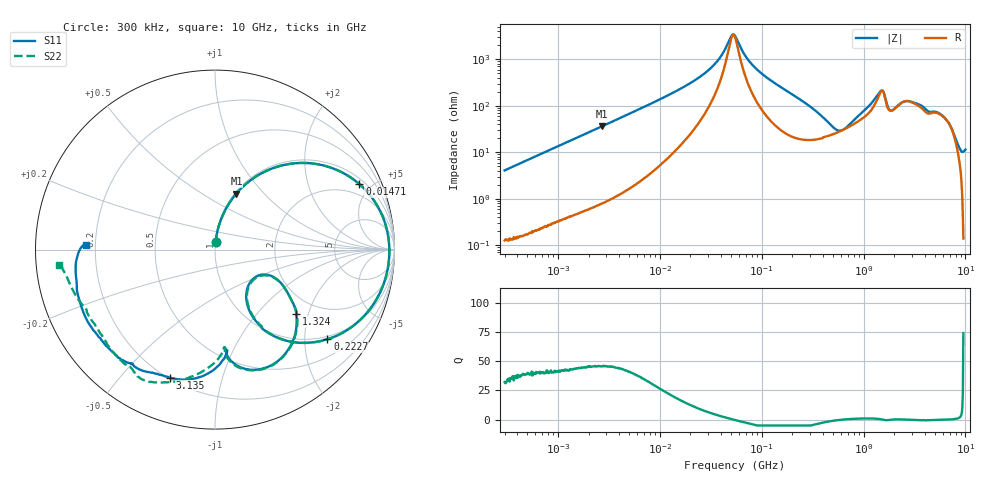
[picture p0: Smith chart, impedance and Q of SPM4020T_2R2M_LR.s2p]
! S-Parameter Data Generated by TDK Corporation
! Copyright(C) 2019 TDK Corporation.
! All Rights Reserved.
! TDK P/N: SPM4020T-2R2M-LR (Inductor)
! Property: L=2.2uH at 100kHz
! Size(LxWxT): 4.4x4.1x2mm
! Model Type: s2p (Touchstone File Format Version 1.0)
! Frequency: DC=Yes Start=0.3MHz Stop=10000MHz 802points Log-sweep
! Model Generated on Sep. 23, 2019
! Port Assignments:
!  1 ---@@@--- 2
! Applicable Conditions:
!  Temperature = 25 degC
!  DC Bias Current = 0 A
!  Small Signal Operation
! Terms and conditions regarding TDK Simulation Models
! (1)This simulation model is being provided solely for informational purposes. Please refer to the specifications of the products in terms of detailed characteristics of such products.
! (2)In no event shall TDK Corporation of any of its subsidiaries be liable for any loss or damage arising, directly or indirectly,
!  From any information contained in this simulation model, including, but not limited to loss or damages arising from any inaccuracies, omissions or errors in connection with such information.
! (3)Any and all copyrights on this simulation model are owned by TDK Corporation.
!  Duplication or redistribution of this simulation model without prior written permission from TDK Corporation is prohibited.
! (4)This simulation model is subject to any modification or change without any prior notice.
! (5)Neither TDK Corporation nor any of its subsidiaries shall make any warranty, express or implied,
!  Including but not limited to the correctness, implied warranties of merchantability and fitness for a particular purpose with respect to this simulation models.
! (6)The use of this simulation model shall be deemed to have consented to the terms and conditions hereof.
# Hz S MA R 50
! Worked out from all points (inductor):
!   801 points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, 300 kHz to 10 GHz, reference 50 ohm
!   read as one part in series: L = 2.15 uH near 318.3 kHz
!   highest Q = 45.7 at 2.696 MHz (marker M1), where L = 2.12 uH
!   self-resonance near 52.78 MHz
!   S11 on the Smith chart (normalised r, x): 300 kHz: 1.00, +0.08; 14.71 MHz: 1.28, +4.27; 222.7 MHz: 0.92, -2.57; 1.324 GHz: 1.56, -1.68; 3.135 GHz: 0.21, -0.69; 10 GHz: 0.16, +0.02
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300000  0.04023 86.0  0.9979 -2.3  0.9979 -2.3  0.04006 85.8
1713600  0.2213 75.9  0.9702 -12.8  0.9702 -12.8  0.2213 75.9
2695816  0.3345 69.1  0.9351 -19.6  0.935 -19.6  0.3345 69.1
9671944  0.7823 36.1  0.5949 -51.8  0.5949 -51.8  0.7822 36.1
1.470778e7  0.8836 24.4  0.422 -62.5  0.422 -62.5  0.8837 24.4
3.118733e7  0.962 7.6  0.1543 -72.6  0.1543 -72.6  0.962 7.6
5.051192e7  0.9716 -1.2  0.03085 -24.6  0.03087 -24.6  0.9716 -1.2
5.477226e7  0.9713 -2.7  0.03048 17.1  0.03047 17.1  0.9713 -2.7
8.974917e7  0.9569 -12.3  0.1575 66.4  0.1575 66.3  0.957 -12.3
2.22675e8  0.801 -38.6  0.5063 44.2  0.5062 44.2  0.801 -38.6
3.126428e8  0.6508 -51.5  0.6479 27.9  0.6479 27.9  0.6509 -51.5
4.807079e8  0.3926 -60.6  0.7522 2.4  0.7522 2.4  0.3939 -60.1
6.821612e8  0.2666 -41.1  0.7349 -20.5  0.7349 -20.5  0.2717 -40.7
1.001841e9  0.3883 -25.8  0.5963 -47.1  0.5963 -47.1  0.3976 -26.4
1.323741e9  0.5781 -38.4  0.3779 -62.5  0.3779 -62.5  0.5937 -39.4
1.525386e9  0.7064 -57.9  0.2573 -49.2  0.2573 -49.3  0.7146 -60.2
1.767019e9  0.625 -81.9  0.4036 -39.7  0.4036 -39.7  0.6055 -83.5
2.38587e9  0.644 -88.0  0.2986 -70.0  0.2987 -70.0  0.6314 -90.3
3.135132e9  0.7567 -109.5  0.2303 -69.0  0.2303 -69.0  0.7698 -107.0
6.333834e9  0.8079 -137.7  0.1958 -95.7  0.1959 -95.8  0.7944 -141.8
8.211115e9  0.7949 -165.6  0.1594 -118.9  0.1594 -119.1  0.8278 -165.9
1e10  0.7182 177.9  0.1197 -129.3  0.1198 -129.5  0.8741 -174.3
